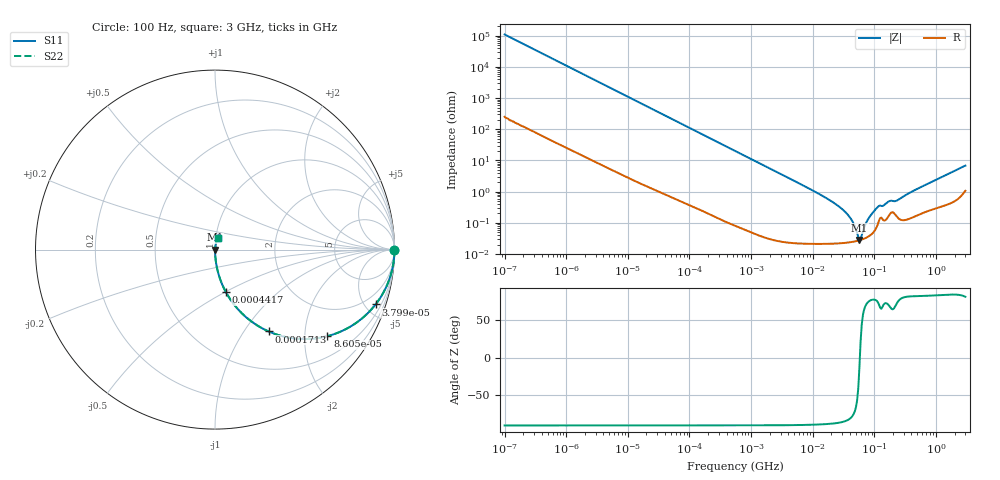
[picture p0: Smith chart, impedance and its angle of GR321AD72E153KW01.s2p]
!Murata Part Number: GR321AD72E153KW01
!These Parameters are Measured in Series Mode Connection
!Data Generated on Mar 13, 2026
!  o--ll--o
!Port1  Port2
!  o------o
!Operation Temp=25[degC], DC Bias Voltage=0[V]
!Freq. Start=100[Hz] Stop=3[GHz] 401[Steps]
# Hz S RI R 50
!Freq.(Hz) S11(Real) S11(Imag) S21(Real) S21(Imag) S12(Real) S12(Imag) S22(Real) S22(Imag)
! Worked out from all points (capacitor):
!   401 points, 100 Hz to 3 GHz, reference 50 ohm
!   read as one part in series: C = 14.4 nF near 109 Hz
!   lowest |Z| = 28.2 mohm at 57.2 MHz (marker M1)
!   series resonance near 58.12 MHz, so ESL is about 520 pH
!   S11 on the Smith chart (normalised r, x): 100 Hz: open; 37.98 kHz: 1.02, -5.86; 86.05 kHz: 1.01, -2.59; 171.3 kHz: 1.00, -1.30; 441.7 kHz: 1.00, -0.51; 3 GHz: 1.02, +0.13
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100  1 -0.000907  2.9e-06 0.000907  2.9e-06 0.000907  1 -0.000907
1788  0.9997 -0.0162  0.000299 0.0162  0.000299 0.0162  0.9997 -0.0162
10003  0.9917 -0.0894  0.00828 0.0894  0.00828 0.0894  0.9917 -0.0894
31977  0.9229 -0.2653  0.0771 0.2653  0.0771 0.2653  0.9229 -0.2653
37985  0.8948 -0.3053  0.1052 0.3053  0.1052 0.3053  0.8948 -0.3053
86054  0.6258 -0.4823  0.3742 0.4823  0.3742 0.4823  0.6258 -0.4823
171338  0.2983 -0.4558  0.7017 0.4558  0.7017 0.4558  0.2983 -0.4558
441669  0.061 -0.2374  0.939 0.2374  0.939 0.2374  0.061 -0.2374
547723  0.0407 -0.1957  0.9593 0.1957  0.9593 0.1957  0.0407 -0.1957
1750920  0.00439 -0.0637  0.9956 0.0637  0.9956 0.0637  0.00439 -0.0637
9794414  0.000335 -0.0111  0.9997 0.0111  0.9997 0.0111  0.000335 -0.0111
2.035898e7  0.000237 -0.00484  0.9998 0.00484  0.9998 0.00484  0.000237 -0.00484
3.268714e7  0.000232 -0.00236  0.9998 0.00236  0.9998 0.00236  0.000232 -0.00236
4.231884e7  0.000243 -0.00126  0.9998 0.00126  0.9998 0.00126  0.000243 -0.00126
5.719833e7  0.000275 -6.22e-05  0.9997 6.22e-05  0.9997 6.22e-05  0.000275 -6.22e-05
6.234031e7  0.00029 0.000277  0.9997 -0.000277  0.9997 -0.000277  0.00029 0.000277
7.730952e7  0.000351 0.00116  0.9996 -0.00116  0.9996 -0.00116  0.000351 0.00116
1.000898e8  0.000549 0.00238  0.9995 -0.00238  0.9995 -0.00238  0.000549 0.00238
1.138854e8  0.000914 0.00311  0.9991 -0.00311  0.9991 -0.00311  0.000914 0.00311
1.751444e8  0.00183 0.00462  0.9982 -0.00462  0.9982 -0.00462  0.00183 0.00462
2.36726e8  0.00152 0.00506  0.9985 -0.00506  0.9985 -0.00506  0.00152 0.00506
3e9  0.0149 0.0658  0.9851 -0.0658  0.9851 -0.0658  0.0149 0.0658
